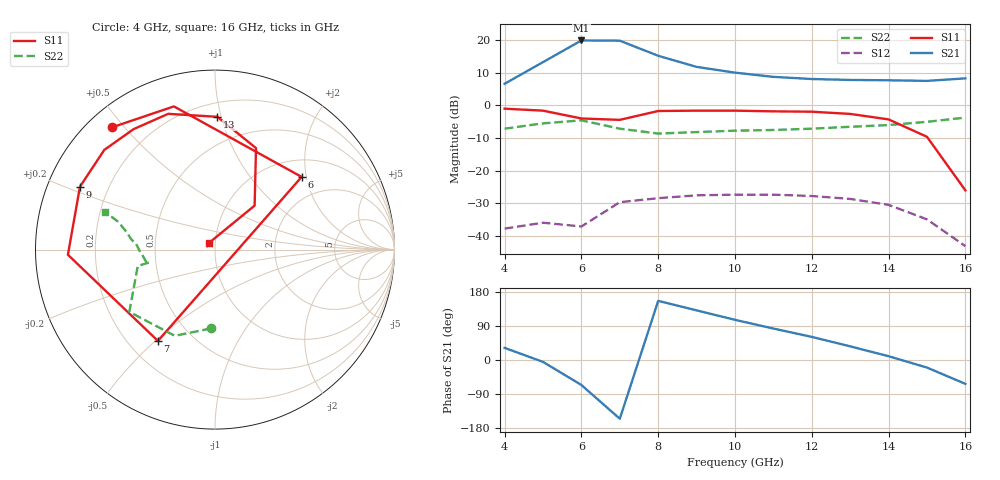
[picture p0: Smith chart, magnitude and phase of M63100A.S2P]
!  MGA-63100 S PARAMETERS
!  Vd=10V  Id=140mA  LAST UPDATED 07-22-92
# ghz s ma r 50
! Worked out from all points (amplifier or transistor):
!   13 points, 4 GHz to 16 GHz, reference 50 ohm
!   highest |S21| = 19.9 dB at 6 GHz (marker M1)
!   |S21| within 3 dB of that: 5.548 GHz to 7.634 GHz (2.086 GHz wide, 31.7 % of centre)
!   unconditionally stable (mu >= 1): start of sweep to 7.466 GHz; 8.379 GHz to end of sweep
!   at 6 GHz: K = 1.81, MAG = 23.3 dB, |S12| = -37.1 dB
!   at 10 GHz: K = 1.31, MAG = 15.3 dB, |S12| = -27.3 dB
!   at 16 GHz: K = 15.86, MAG = 10.7 dB, |S12| = -43.1 dB
!   S11 on the Smith chart (normalised r, x): 4 GHz: 0.07, +0.46; 6 GHz: 1.40, +1.88; 7 GHz: 0.32, -0.51; 9 GHz: 0.10, +0.22; 13 GHz: 0.30, +0.97; 16 GHz: 0.93, +0.07
4  0.89 130.0  2.14 32.0  0.013 96.0  0.44 -93.0
5  0.83 106.0  4.59 -5.0  0.016 90.0  0.53 -115.0
6  0.63 40.0  9.85 -66.0  0.014 110.0  0.59 -144.0
7  0.6 -122.0  9.77 -155.0  0.033 108.0  0.44 -168.0
8  0.82 -178.0  5.74 156.0  0.038 94.0  0.37 -169.0
9  0.83 155.0  3.88 131.0  0.042 79.0  0.39 -170.0
10  0.83 138.0  3.17 106.0  0.043 65.0  0.41 -177.0
11  0.81 124.0  2.73 83.0  0.043 59.0  0.42 -179.0
12  0.8 109.0  2.53 61.0  0.041 48.0  0.44 176.0
13  0.74 89.0  2.45 36.0  0.037 35.0  0.47 173.0
14  0.61 68.0  2.42 10.0  0.03 18.0  0.5 169.0
15  0.33 48.0  2.37 -20.0  0.018 11.0  0.56 164.0
16  0.05 134.0  2.59 -63.0  0.007 13.0  0.65 161.0
